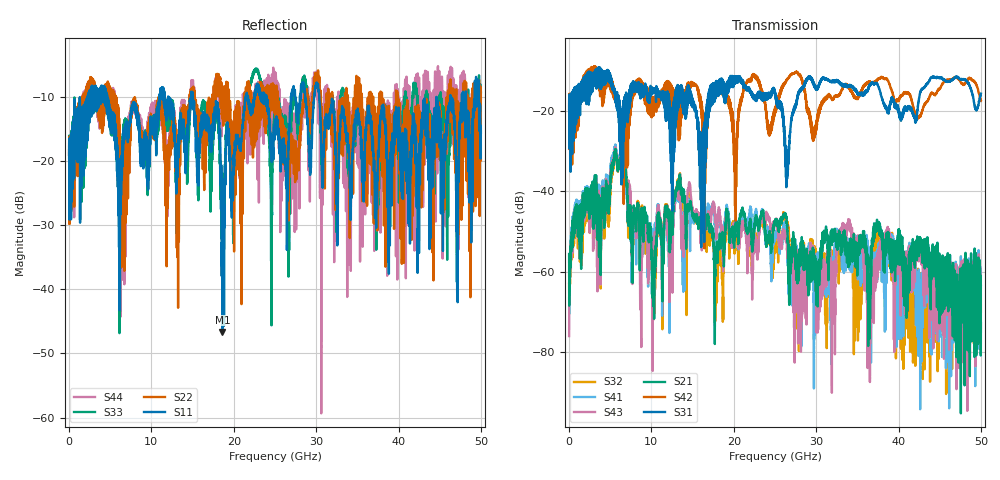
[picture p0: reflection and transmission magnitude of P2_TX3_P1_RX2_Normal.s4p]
!Keysight Technologies,N5225B,MY57041031,A.13.20.10
!Date: Friday, May 31, 2019 11:16:24
!Correction: S11(Full 4 Port(1,2,3,4))
!S12(Full 4 Port(1,2,3,4))
!S13(Full 4 Port(1,2,3,4))
!S14(Full 4 Port(1,2,3,4))
!S21(Full 4 Port(1,2,3,4))
!S22(Full 4 Port(1,2,3,4))
!S23(Full 4 Port(1,2,3,4))
!S24(Full 4 Port(1,2,3,4))
!S31(Full 4 Port(1,2,3,4))
!S32(Full 4 Port(1,2,3,4))
!S33(Full 4 Port(1,2,3,4))
!S34(Full 4 Port(1,2,3,4))
!S41(Full 4 Port(1,2,3,4))
!S42(Full 4 Port(1,2,3,4))
!S43(Full 4 Port(1,2,3,4))
!S44(Full 4 Port(1,2,3,4))
!S4P File: Measurements: <S11,S12,S13,S14>,
!<S21,S22,S23,S24>,
!<S31,S32,S33,S34>,
!<S41,S42,S43,S44>:
# Hz S  dB  R 50.0
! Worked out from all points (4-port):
!   5000 points, 10 MHz to 50 GHz, reference 50 ohm
!   strongest paths, dB at 10 MHz, 12.51 GHz, 25.01 GHz, 37.51 GHz, 50 GHz:
!     S31: -19.5, -43.4, -16.0, -13.6, -15.6
!     S42: -19.4, -16.3, -19.1, -12.0, -17.4
!     S21: -55.6, -49.9, -47.7, -48.1, -72.8
!     S43: -76.1, -58.7, -47.4, -58.6, -74.1
!     S41: -66.6, -63.6, -51.4, -54.9, -63.5
!     S32: -63.0, -48.7, -52.3, -50.2, -69.9
!   lowest |S11| = -46.6 dB at 18.62 GHz (marker M1), VSWR 1.01, Z = 49.6 - j0.268 ohm
!   |S11| at or under -10 dB: 4.63 GHz to 10.95 GHz (6.318 GHz wide, 81.1 % of centre); 15.04 GHz to 21.46 GHz (6.427 GHz wide, 35.2 % of centre); 30.38 GHz to 44.61 GHz (14.23 GHz wide, 37.9 % of centre)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
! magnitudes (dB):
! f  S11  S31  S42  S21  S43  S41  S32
! 10 MHz  -19.6  -19.5  -19.4  -55.6  -76.1  -66.6  -63.0
! 5.57 GHz  -15.2  -15.7  -17.2  -30.0  -29.6  -28.8  -30.6
! 8.77 GHz  -19.5  -14.4  -14.2  -44.4  -78.8  -56.8  -44.5
! 18.62 GHz  -46.6  -12.2  -15.5  -50.8  -53.1  -52.4  -61.3
! 26.48 GHz  -22.3  -36.8  -12.2  -48.3  -54.9  -51.3  -48.3
! 29.13 GHz  -18.7  -11.3  -20.6  -56.6  -59.0  -55.7  -58.2
! 50 GHz  -15.6  -15.6  -17.4  -72.8  -74.1  -63.5  -69.9
